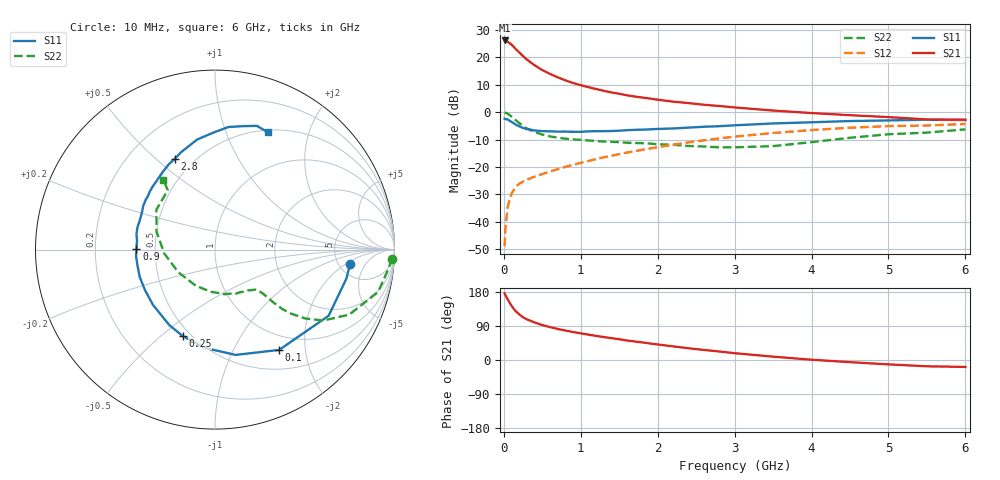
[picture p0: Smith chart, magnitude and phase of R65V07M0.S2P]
! SIEMENS Small Signal Semiconductors
! BFR193
! Si NPN RF Bipolar Junction Transistor in SOT23
! VCE = 5 V  IC = 7 mA
! Common Emitter S-Parameters:  May  1996
# GHz  S  MA  R  50
!  f  S11  S21  S12  S22
! GHz  MAG  ANG  MAG  ANG  MAG  ANG  MAG  ANG
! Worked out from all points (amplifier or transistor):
!   36 points, 10 MHz to 6 GHz, reference 50 ohm
!   highest |S21| = 26.1 dB at 10 MHz (marker M1)
!   |S21| within 3 dB of that: start of sweep to 149.7 MHz
!   unconditionally stable (mu >= 1): 830.3 MHz to 2.004 GHz
!   at 250 MHz: K = 0.53, MSG = 22.9 dB, |S12| = -25.3 dB
!   at 1.4 GHz: K = 1.05, MAG = 10.1 dB, |S12| = -15.9 dB
!   at 6 GHz: K = 0.95, MSG = 0.8 dB, |S12| = -4.3 dB
!   lowest NFmin = 1.20 dB at 450 MHz
!   S11 on the Smith chart (normalised r, x): 10 MHz: 6.25, -2.43; 100 MHz: 0.77, -1.54; 250 MHz: 0.45, -0.59; 900 MHz: 0.39, +0.01; 2.8 GHz: 0.40, +0.58; 6 GHz: 0.53, +1.41
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0.01  0.7565 -6.3  20.24 175.9  0.0036 87.5  0.9871 -2.9
0.02  0.7498 -12.4  19.96 171.5  0.0075 83.5  0.9735 -6.1
0.05  0.7327 -30.2  19.22 159.9  0.0188 75.5  0.9392 -14.5
0.1  0.6634 -57.4  17 143.0  0.0327 65.1  0.8316 -25.8
0.15  0.5979 -78.9  14.31 129.8  0.0427 57.9  0.7203 -33.3
0.2  0.5504 -96.0  12.22 120.3  0.0495 54.3  0.631 -37.4
0.25  0.5141 -110.5  10.46 112.7  0.0542 52.2  0.5561 -40.0
0.3  0.4918 -121.1  9.067 107.2  0.0587 52.0  0.5032 -41.4
0.4  0.463 -138.3  7.141 99.1  0.0666 52.2  0.4347 -42.2
0.5  0.4505 -150.1  5.833 92.2  0.0744 53.4  0.3895 -42.3
0.6  0.4464 -159.9  4.965 86.8  0.0828 55.4  0.3605 -42.6
0.7  0.441 -168.3  4.31 81.9  0.0911 56.5  0.3423 -43.1
0.9  0.4376 179.3  3.393 73.9  0.1098 58.5  0.3185 -44.6
1.1  0.4463 168.7  2.849 66.9  0.1286 60.0  0.3041 -47.9
1.3  0.449 160.1  2.445 60.5  0.1502 60.4  0.2911 -51.5
1.6  0.4685 148.5  2.026 51.5  0.1828 60.0  0.2767 -58.8
2.2  0.5033 129.9  1.552 36.0  0.2546 56.0  0.254 -78.2
2.8  0.5537 113.8  1.293 22.4  0.3315 49.1  0.2278 -106.4
3.5  0.6215 99.2  1.068 8.8  0.4158 38.8  0.2401 -148.2
4.5  0.6872 83.7  0.879 -5.7  0.5195 23.1  0.3405 163.0
5.5  0.7279 71.3  0.736 -16.6  0.5695 6.8  0.4227 128.5
6  0.7168 65.7  0.726 -18.3  0.6078 2.0  0.4851 126.4
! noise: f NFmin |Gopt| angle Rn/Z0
0.45  1.2  0.24  125  0.12
0.9  1.25  0.36  154  0.11
1.8  2  0.55  -156  0.13
